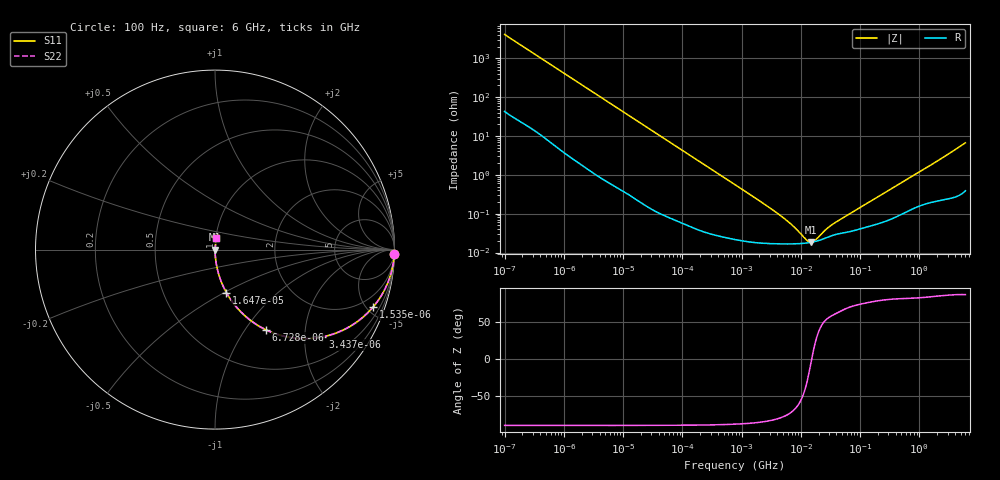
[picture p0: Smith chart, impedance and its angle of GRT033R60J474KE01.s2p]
!Murata Part Number: GRT033R60J474KE01
!These Parameters are Measured in Series Mode Connection
!Data Generated on Jun 19, 2026
!  o--ll--o
!Port1  Port2
!  o------o
!Operation Temp=25[degC], DC Bias Voltage=0[V]
!Freq. Start=100[Hz] Stop=6[GHz] 401[Steps]
# Hz S RI R 50
!Freq.(Hz) S11(Real) S11(Imag) S21(Real) S21(Imag) S12(Real) S12(Imag) S22(Real) S22(Imag)
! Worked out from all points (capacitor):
!   401 points, 100 Hz to 6 GHz, reference 50 ohm
!   read as one part in series: C = 386 nF near 109 Hz
!   lowest |Z| = 18.3 mohm at 14.88 MHz (marker M1)
!   series resonance near 15.28 MHz, so ESL is about 280 pH
!   S11 on the Smith chart (normalised r, x): 100 Hz: 2, -82; 1.535 kHz: 1.05, -5.45; 3.437 kHz: 1.02, -2.44; 6.728 kHz: 1.01, -1.25; 16.47 kHz: 1.00, -0.51; 6 GHz: 1.01, +0.13
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100  0.9992 -0.0243  0.000843 0.0243  0.000843 0.0243  0.9992 -0.0243
479  0.9858 -0.1135  0.0142 0.1135  0.0142 0.1135  0.9858 -0.1135
938  0.9501 -0.2132  0.0499 0.2132  0.0499 0.2132  0.9501 -0.2132
1535  0.8792 -0.3216  0.1208 0.3216  0.1208 0.3216  0.8792 -0.3216
2008  0.8111 -0.3872  0.1889 0.3872  0.1889 0.3872  0.8111 -0.3872
3437  0.5981 -0.4862  0.4019 0.4862  0.4019 0.4862  0.5981 -0.4862
4702  0.4449 -0.4928  0.5551 0.4928  0.5551 0.4928  0.4449 -0.4928
6728  0.2834 -0.4464  0.7166 0.4464  0.7166 0.4464  0.2834 -0.4464
10527  0.1409 -0.3435  0.8591 0.3435  0.8591 0.3435  0.1409 -0.3435
16473  0.0639 -0.2401  0.9361 0.2401  0.9361 0.2401  0.0639 -0.2401
40335  0.012 -0.1041  0.988 0.1041  0.988 0.1041  0.012 -0.1041
129199  0.00157 -0.0331  0.9984 0.0331  0.9984 0.0331  0.00157 -0.0331
774597  0.000247 -0.00558  0.9998 0.00558  0.9998 0.00558  0.000247 -0.00558
4440638  0.000168 -0.000901  0.9998 0.000901  0.9998 0.000901  0.000168 -0.000901
7266822  0.000167 -0.000466  0.9998 0.000466  0.9998 0.000466  0.000167 -0.000466
1.243624e7  0.000175 -0.000118  0.9998 0.000118  0.9998 0.000118  0.000175 -0.000118
1.487547e7  0.000182 -1.52e-05  0.9998 1.52e-05  0.9998 1.52e-05  0.000182 -1.52e-05
1.555665e7  0.000185 1.03e-05  0.9998 -1.03e-05  0.9998 -1.03e-05  0.000185 1.03e-05
1.779312e7  0.000193 8.61e-05  0.9998 -8.61e-05  0.9998 -8.61e-05  0.000193 8.61e-05
3.482834e7  0.000277 0.000463  0.9997 -0.000463  0.9997 -0.000463  0.000277 0.000463
3.124326e8  0.000708 0.00403  0.9993 -0.00403  0.9993 -0.00403  0.000708 0.00403
6e9  0.00823 0.0657  0.9918 -0.0657  0.9918 -0.0657  0.00823 0.0657
